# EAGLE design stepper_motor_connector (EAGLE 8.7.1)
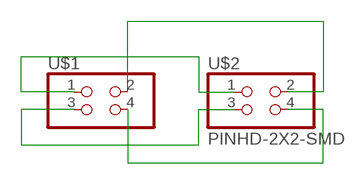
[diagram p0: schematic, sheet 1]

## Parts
U$1  PINHD-2X2-SMD  [2X02SMD]
U$2  PINHD-2X2-SMD  [2X02SMD]

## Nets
N$1: U$1.1 U$2.1
N$2: U$1.2 U$2.2
N$3: U$1.3 U$2.3
N$4: U$1.4 U$2.4

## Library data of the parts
U$1 U$2 = fab:PINHD-2X2-SMD

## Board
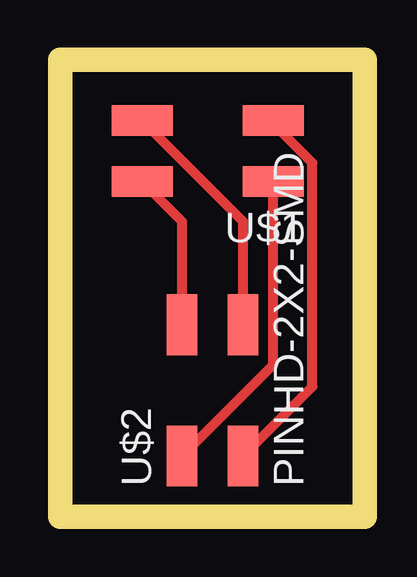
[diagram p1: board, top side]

Size 12.37 x 19.04 mm. Coordinates in mm from the lower left corner, seen from the top.
Outline: 0,0 12.37,0 12.37,19.04 0,19.04 0,0
Copper layers (1*16): Top 0.035mm / dielectric 1.5mm / Bottom 0.035mm
Design rules "default": minimum track width 6mil, minimum drill 0.35mm, track to track 6mil, track to pad 6mil, pad to pad 6mil, via to via 6mil, smd to smd 6mil, copper to edge 40mil, drill to drill 6mil, minimum pad ring 10mil, minimum via ring 8mil, stop-mask expansion 4mil, vias tented up to drill 0mil, thermal gap 10mil
Milling: 4 lines

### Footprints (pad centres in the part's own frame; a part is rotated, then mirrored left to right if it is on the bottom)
2X02SMD = smd 2.54 x 1.27: 1 -2.54,1.27; 2 2.92,1.27; 3 -2.54,-1.27; 4 2.92,-1.27

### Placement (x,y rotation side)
U$1  6.35,15.24 180 top
U$2  6.35,5.08 90 top

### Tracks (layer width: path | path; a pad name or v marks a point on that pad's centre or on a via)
N$1
  Top 0.406: U$2.1 8.89,6.35 U$1.1
N$2
  Top 0.406: U$1.2 5.08,12.32 U$2.2
N$3
  Top 0.406: U$1.3 8.89,16.38 10.52,14.75 10.52,5.44 U$2.3
N$4
  Top 0.406: U$1.4 7.62,12.32 U$2.4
